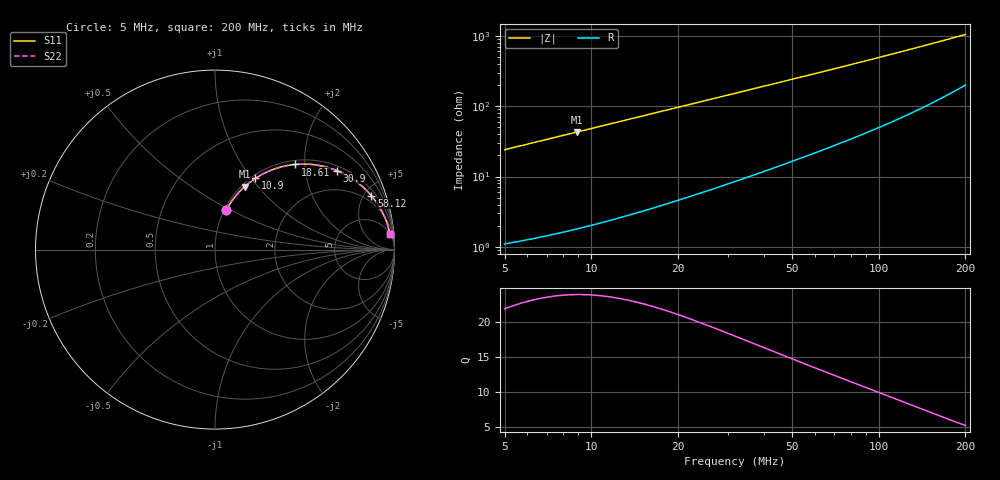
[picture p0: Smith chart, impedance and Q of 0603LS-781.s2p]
# MHz S MA R 50
!Freq  MagS11  AngS11  MagS21  AngS21  MagS12  AngS12  MagS22  AngS22
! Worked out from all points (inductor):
!   801 points, 5 MHz to 200 MHz, reference 50 ohm
!   read as one part in series: L = 765 nH near 5.093 MHz
!   highest Q = 23.8 at 8.898 MHz (marker M1), where L = 765 nH
!   S11 on the Smith chart (normalised r, x): 5 MHz: 1.02, +0.48; 10.9 MHz: 1.04, +1.05; 18.61 MHz: 1.08, +1.79; 30.9 MHz: 1.16, +2.97; 58.12 MHz: 1.41, +5.62; 200 MHz: 5, +21
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5  0.2314 74.0  0.9623 -13.4  0.9623 -13.4  0.2314 74.0
5.957552  0.2723 71.7  0.9504 -15.8  0.9504 -15.8  0.2723 71.7
6.809928  0.3073 69.7  0.9386 -17.9  0.9386 -17.9  0.3073 69.7
7.820235  0.3472 67.3  0.9233 -20.3  0.9233 -20.3  0.3472 67.3
8.897989  0.3875 64.8  0.9058 -22.8  0.9058 -22.8  0.3875 64.8
10.89946  0.4563 60.5  0.8708 -27.1  0.8708 -27.1  0.4563 60.5
12.63245  0.5095 56.9  0.8389 -30.6  0.8389 -30.6  0.5095 56.9
14.50657  0.5606 53.4  0.8038 -34.1  0.8038 -34.1  0.5606 53.4
18.60818  0.6519 46.7  0.7285 -40.6  0.7285 -40.6  0.6519 46.7
21.56683  0.7031 42.6  0.6777 -44.6  0.6777 -44.6  0.7031 42.6
24.53909  0.7447 39.0  0.6307 -48.0  0.6307 -48.0  0.7447 39.0
27.66466  0.78 35.8  0.5858 -51.2  0.5858 -51.2  0.78 35.8
30.90204  0.8095 32.9  0.5441 -53.9  0.5441 -53.9  0.8095 32.9
37.50553  0.8537 28.1  0.4722 -58.4  0.4722 -58.4  0.8537 28.1
46.79709  0.8929 23.2  0.3951 -63.0  0.3951 -63.0  0.8929 23.2
58.12191  0.9212 19.0  0.3272 -66.7  0.3272 -66.7  0.9212 19.0
70.21752  0.9394 15.9  0.2751 -69.4  0.2751 -69.4  0.9394 15.9
85.61625  0.9532 13.1  0.2276 -71.7  0.2276 -71.7  0.9532 13.1
102.9578  0.9625 10.9  0.1896 -73.2  0.1896 -73.2  0.9625 10.9
135.1485  0.9716 8.2  0.1432 -74.5  0.1432 -74.5  0.9716 8.2
167.8542  0.9759 6.4  0.1135 -74.6  0.1135 -74.6  0.9759 6.4
200  0.978 5.3  0.09342 -73.8  0.09342 -73.8  0.978 5.3
